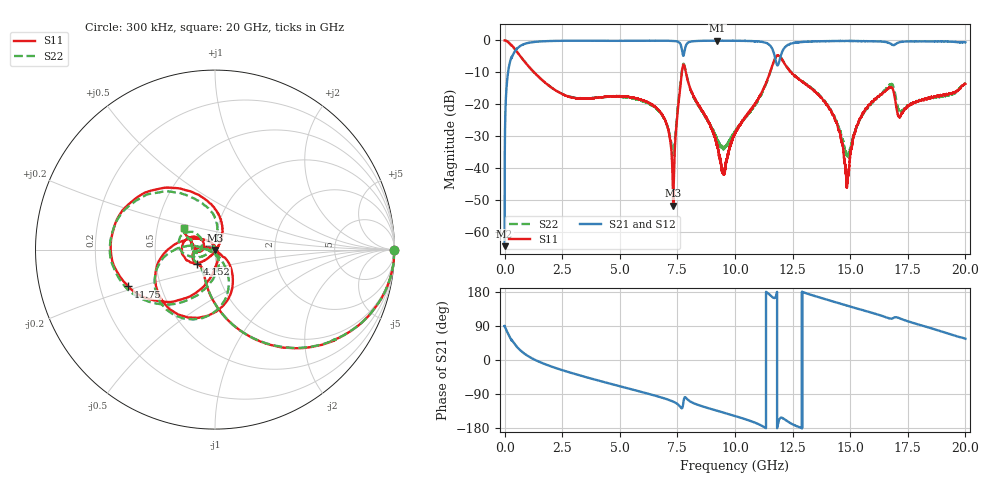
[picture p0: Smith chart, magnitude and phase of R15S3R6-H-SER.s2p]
!{R15S3R6}
!Johanson Technology Inc.
!www.johansontechnology.com
!Test Board Conditions:
!Substrate Type  RO4350B
!Substrate Thickness  20 mil
!Substrate Dk  3.66
!TL Type: GCPW
!TL Trace Width  34 mil
!TL Gap  10 mil
!Electrode orientation  Horizontal
!DUT TOPOLOGY	SERIES
!Mounting Pad LxW  26x52 mil
! Created Sat Feb  6 13:54:50 2021
# hz S ma R 50
! 2 Port Network Data from SP1.SP block
! freq  magS11  angS11  magS21  angS21  magS12  angS12  magS22  angS22
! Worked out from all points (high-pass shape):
!   20001 points, 300 kHz to 20 GHz, reference 50 ohm
!   highest |S21| = -0.07 dB at 9.239 GHz (marker M1); lowest = -64.6 dB at 300 kHz (marker M2)
!   |S21| within 3 dB of the highest: 477.5 MHz to 7.704 GHz (7.226 GHz wide, 177 % of centre); 12.08 GHz to end of sweep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
!   lowest |S11| = -51.9 dB at 7.318 GHz (marker M3), VSWR 1.01, Z = 49.8 - j0.196 ohm
!   |S11| at or under -10 dB: 1.28 GHz to 7.695 GHz (6.415 GHz wide, 143 % of centre); 7.868 GHz to 11.52 GHz (3.653 GHz wide, 37.7 % of centre); 12.43 GHz to end of sweep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
!   |S22| runs from -36.6 to 0.0 dB; largest |S21 - S12| = 0.015
!   S11 on the Smith chart (normalised r, x): 300 kHz: open; 4.152 GHz: 0.81, -0.13; 11.75 GHz: 0.32, -0.18; 20 GHz: 0.69, +0.17
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300000  1 -0.3  0.0005914 89.4  0.0006886 90.3  0.9972 -0.2
1.183e8  0.9657 -16.4  0.2539 73.3  0.2545 73.3  0.966 -16.4
3.753e8  0.788 -42.6  0.6105 47.2  0.6116 47.3  0.788 -42.5
1.2703e9  0.319 -88.0  0.9459 1.9  0.9444 1.8  0.3185 -88.0
3.3343e9  0.1225 -129.1  0.9896 -41.8  0.9892 -41.9  0.1239 -133.3
4.1523e9  0.1276 -142.3  0.9878 -55.6  0.9875 -55.5  0.1279 -147.7
6.6673e9  0.08191 169.4  0.9891 -96.5  0.9896 -96.5  0.08037 178.5
7.3183e9  0.00255 -129.6  0.9836 -109.8  0.9839 -109.8  0.01644 -117.4
7.7793e9  0.4154 -130.4  0.597 -104.8  0.5988 -104.7  0.429 -131.9
9.2393e9  0.02142 97.0  0.9919 -134.2  0.9897 -134.3  0.02749 -159.7
9.5063e9  0.009017 19.4  0.9909 -138.9  0.9887 -138.9  0.02029 -119.6
1.00003e10  0.03488 -59.8  0.9875 -147.8  0.9881 -147.8  0.03732 -75.6
1.12783e10  0.1875 -103.7  0.9324 -177.4  0.9326 -177.3  0.18 -96.7
1.17463e10  0.5248 -157.0  0.5245 165.1  0.5241 165.1  0.5266 -153.3
1.21153e10  0.4534 131.1  0.7379 -155.0  0.738 -155.4  0.46 136.6
1.33343e10  0.1733 79.4  0.9636 171.2  0.9622 171.3  0.1768 90.3
1.43513e10  0.05522 56.3  0.9805 152.8  0.9788 152.7  0.05868 82.2
1.48683e10  0.005815 -46.7  0.9813 143.5  0.982 143.4  0.01563 142.6
1.54633e10  0.06176 -129.5  0.9798 133.1  0.975 133.1  0.06102 -150.5
1.66673e10  0.178 -168.4  0.9214 110.2  0.9109 110.3  0.1927 -179.7
1.71533e10  0.06255 172.2  0.943 109.8  0.9368 110.0  0.07464 163.9
2e10  0.2088 145.0  0.9373 56.1  0.9311 55.8  0.2135 144.4
